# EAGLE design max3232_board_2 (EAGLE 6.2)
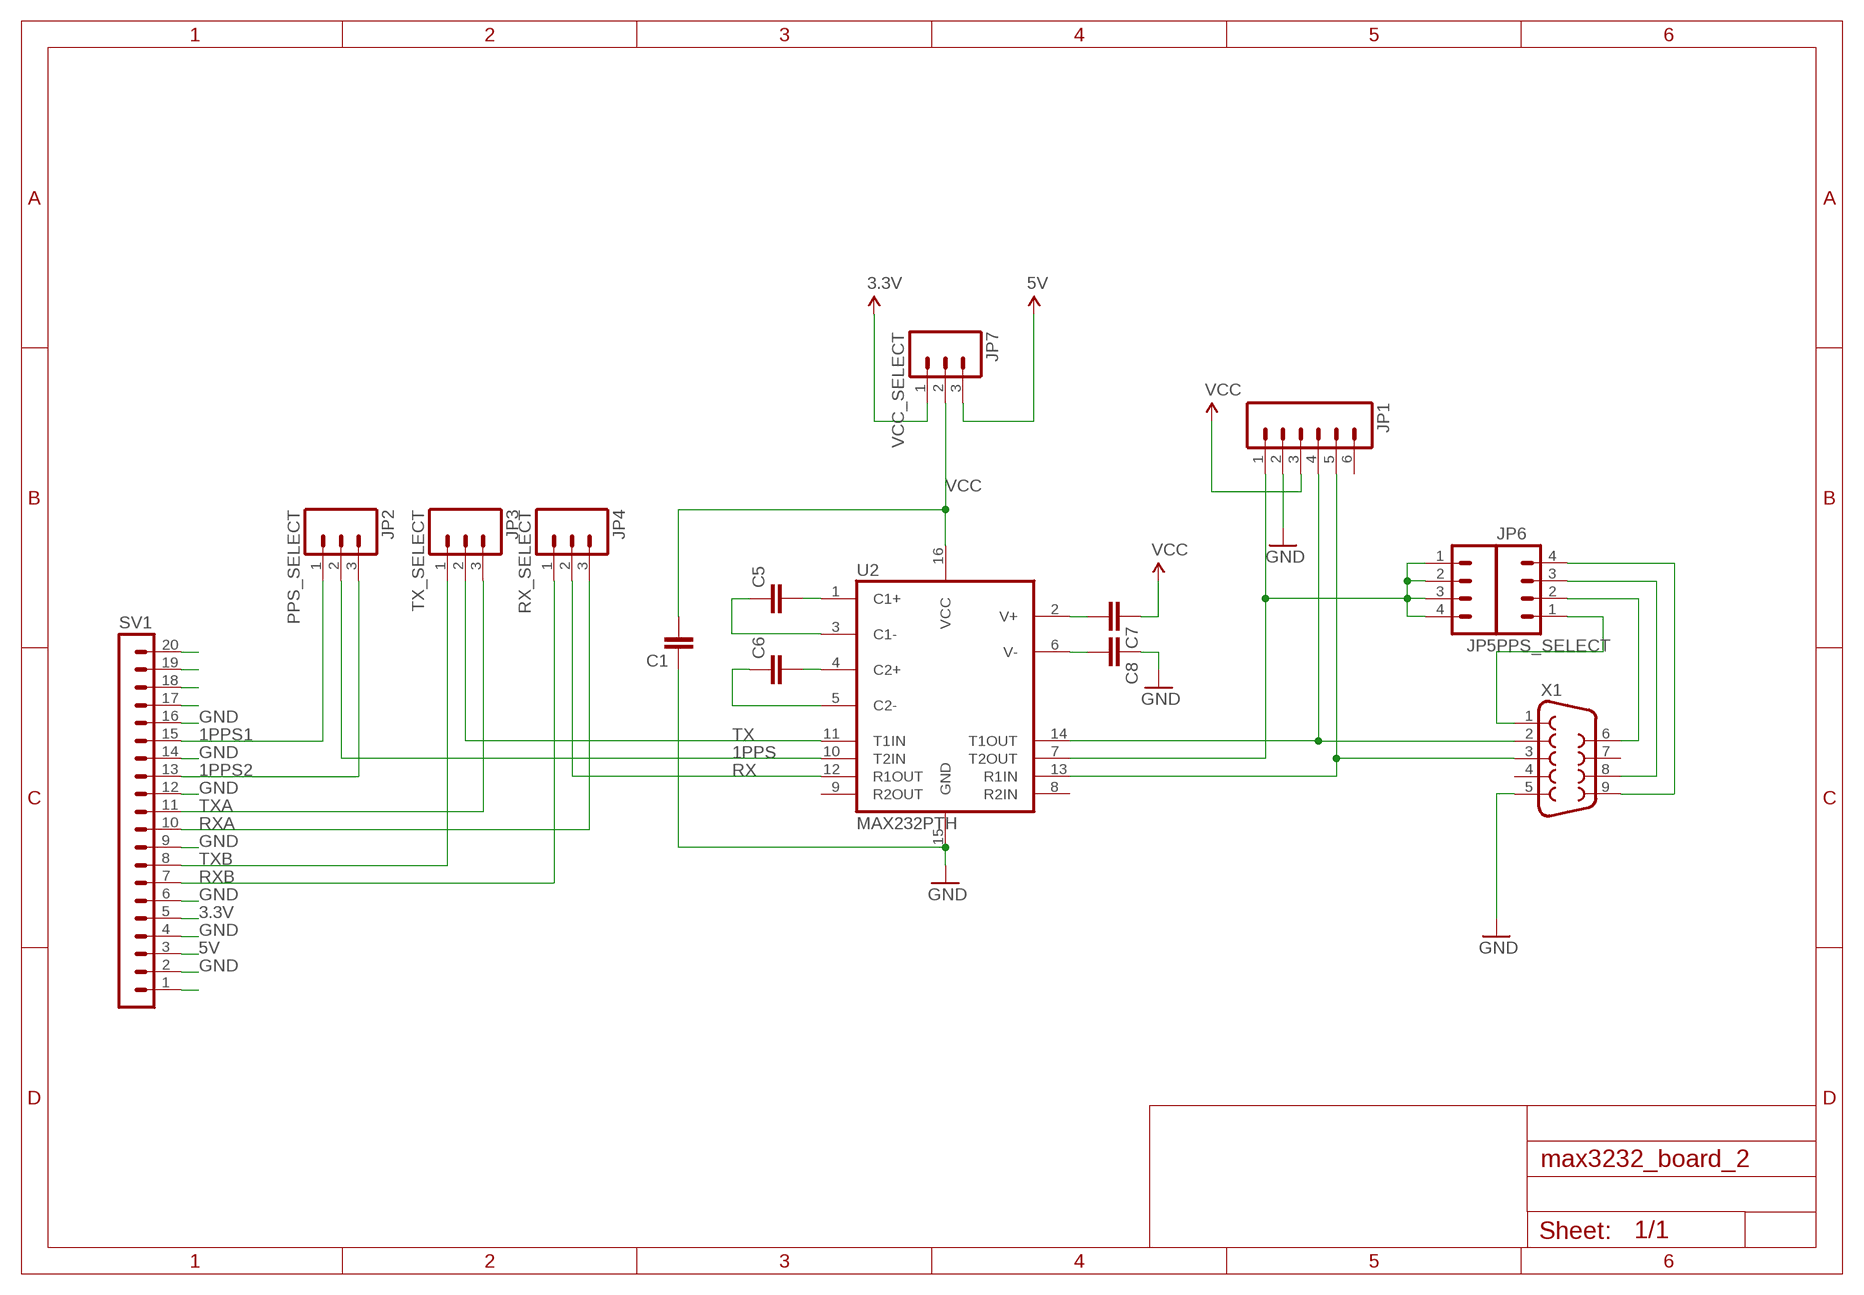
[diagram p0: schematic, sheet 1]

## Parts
C1  CAPPTH1  [CAP-PTH-5MM]
C5  CAPPTH1  [CAP-PTH-5MM]
C6  CAPPTH1  [CAP-PTH-5MM]
C7  CAPPTH1  [CAP-PTH-5MM]
C8  CAPPTH1  [CAP-PTH-5MM]
JP1  M06LONGPADS  [1X06_LONGPADS]
JP2  PPS_SELECT  M03LONGPADS  [1X03_LONGPADS]
JP3  TX_SELECT  M03LONGPADS  [1X03_LONGPADS]
JP4  RX_SELECT  M03LONGPADS  [1X03_LONGPADS]
JP5  M04PTH  [1X04]
JP6  PPS_SELECT  M04PTH  [1X04]
JP7  VСС_SELECT  M03LONGPADS  [1X03_LONGPADS]
SV1  MA20-1W  [MA20-1W]
U2  MAX232PTH  [DIL16]
X1  DB9FEMALE  [DB9]

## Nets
1PPS: JP2.2 U2.10(T2IN)
1PPS1: JP2.1 SV1.15
1PPS2: JP2.3 SV1.13
3.3V: JP7.1 SV1.5
5V: JP7.3 SV1.3
GND: C1.1 C8.1 JP1.2 SV1.2 SV1.4 SV1.6 SV1.9 SV1.12 SV1.14 SV1.16 U2.15(GND) X1.5
N$1: SV1.1
N$6: JP6.1 X1.1
N$7: JP1.4 U2.14(T1OUT) X1.2
N$8: JP1.5 U2.13(R1IN) X1.3
N$10: C6.2 U2.4(C2+)
N$11: C5.2 U2.1(C1+)
N$12: C5.1 U2.3(C1-)
N$13: C6.1 U2.5(C2-)
N$14: C8.2 U2.6(V-)
N$15: C7.2 U2.2(V+)
N$17: SV1.17
N$18: SV1.18
N$19: SV1.19
N$20: SV1.20
N$22: JP1.1 JP5.1 JP5.2 JP5.3 JP5.4 U2.7(T2OUT)
N$23: JP6.2 X1.6
N$24: JP6.3 X1.8
N$25: JP6.4 X1.9
RX: JP4.2 U2.12(R1OUT)
RXA: JP4.3 SV1.10
RXB: JP4.1 SV1.7
TX: JP3.2 U2.11(T1IN)
TXA: JP3.3 SV1.11
TXB: JP3.1 SV1.8
VCC: C1.2 C7.1 JP1.3 JP7.2 U2.16(VCC)
Unconnected: JP1.6 U2.8(R2IN) U2.9(R2OUT) X1.4 X1.7

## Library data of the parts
C1 C5-C8 = SparkFun:CAP: Capacitor
JP1 = SparkFun:M06: Header 6 Standard 6-pin 0.1" header. Use with straight break away headers (SKU : PRT-00116), right angle break away headers (PRT-00553), swiss pins (PRT-00743), machine pins (PRT-00117), and female headers (PRT-00115). Molex polarized connector foot print use with SKU : PRT-08094 with associated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
JP2-JP4 JP7 = SparkFun:M03: Header 3 Standard 3-pin 0.1" header. Use with straight break away headers (SKU : PRT-00116), right angle break away headers (PRT-00553), swiss pins (PRT-00743), machine pins (PRT-00117), and female headers (PRT-00115). Molex polarized connector foot print use with SKU : PRT-08232 with associated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
JP5 JP6 = SparkFun:M04: Header 4 Standard 4-pin 0.1" header. Use with straight break away headers (SKU : PRT-00116), right angle break away headers (PRT-00553), swiss pins (PRT-00743), machine pins (PRT-00117), and female headers (PRT-00115). Molex polarized connector foot print use with SKU : PRT-08231 with associated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
SV1 = con-lstb:MA20-1W: PIN HEADER; OC_FARNELL: unknown; OC_NEWARK: unknown
U2 = SparkFun:MAX232: RS232 Transceiver Very common IC. This is generically called 'MAX232', but works with the 3V equivalent MAX3232 generic ICs. Field tested and mother approved. Spark Fun Electronics SKU : COM-00316 (DIP) and COM-00589 (SMD)
X1 = SparkFun:DB9: DB9 Connector Standard DB9 (D-Sub 9) serial connector. Can be used for CAN bus as well as RS485 and RS232. Footprint production proven. Spark Fun Electronics SKU : PRT-00429

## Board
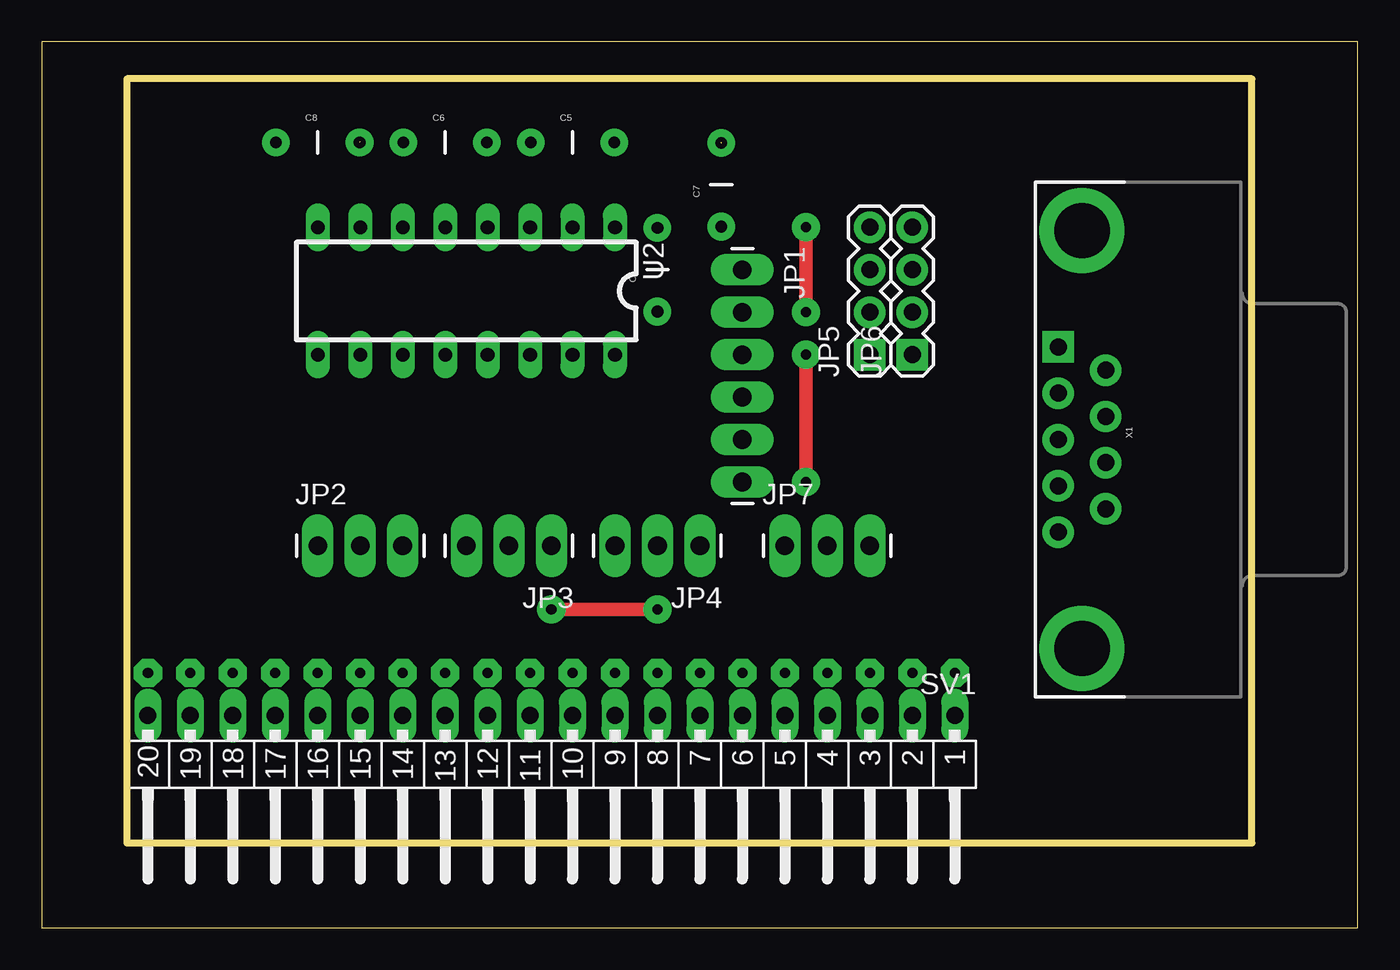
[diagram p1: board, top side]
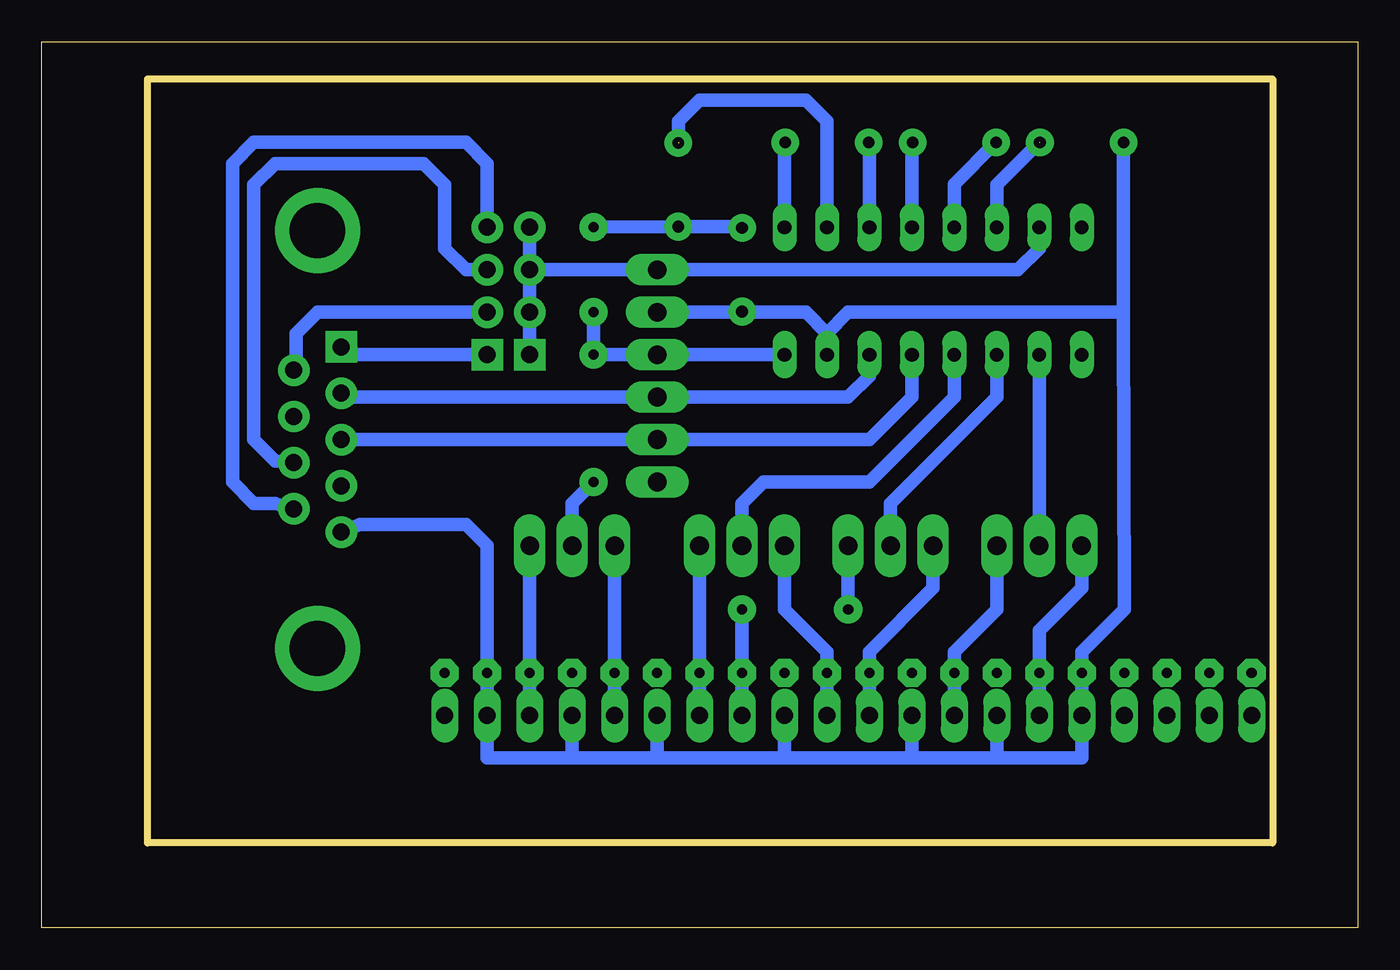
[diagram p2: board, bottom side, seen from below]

Size 78.72 x 53.01 mm. Coordinates in mm from the lower left corner, seen from the top.
Outline: 0,0 78.72,0 78.72,53.01 0,53.01 0,0
Outline: 5.08,5.08 72.39,5.08 72.39,50.8 5.08,50.8 5.08,5.08
Copper layers (1*16): Top 0.035mm / dielectric 1.5mm / Bottom 0.035mm
Design rules: minimum track width 10mil, minimum drill 24mil, track to track 8mil, track to pad 8mil, pad to pad 8mil, via to via 8mil, smd to smd 8mil, copper to edge 40mil, drill to drill 8mil, minimum pad ring 12mil, minimum via ring 12mil, stop-mask expansion 4mil, vias tented up to drill 0mil, thermal gap 10mil

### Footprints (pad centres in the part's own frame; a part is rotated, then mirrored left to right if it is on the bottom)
CAP-PTH-5MM = drill 0.7 pad 1.651: 1 -2.5,0; 2 2.5,0
1X06_LONGPADS = drill 1.118 pad 1.88 long: 1 0,0; 2 2.54,0; 3 5.08,0; 4 7.62,0; 5 10.16,0; 6 12.7,0
1X03_LONGPADS = drill 1.118 pad 1.88 long: 1 0,0; 2 2.54,0; 3 5.08,0
1X04 = drill 1.016 pad 1.88 square: 1 0,0 | drill 1.016 pad 1.88: 2 2.54,0; 3 5.08,0; 4 7.62,0
MA20-1W = drill 1.016 long: 1 -24.13,0; 2 -21.59,0; 3 -19.05,0; 4 -16.51,0; 5 -13.97,0; 6 -11.43,0; 7 -8.89,0; 8 -6.35,0; 9 -3.81,0; 10 -1.27,0; 11 1.27,0; 12 3.81,0; 13 6.35,0; 14 8.89,0; 15 11.43,0; 16 13.97,0; 17 16.51,0; 18 19.05,0; 19 21.59,0; 20 24.13,0
DIL16 = drill 0.813 long: 1 -8.89,-3.81; 2 -6.35,-3.81; 3 -3.81,-3.81; 4 -1.27,-3.81; 5 1.27,-3.81; 6 3.81,-3.81; 7 6.35,-3.81; 8 8.89,-3.81; 9 8.89,3.81; 10 6.35,3.81; 11 3.81,3.81; 12 1.27,3.81; 13 -1.27,3.81; 14 -3.81,3.81; 15 -6.35,3.81; 16 -8.89,3.81
DB9 = drill 1.016 pad 1.88 square: 1 -5.54,-1.42 | drill 1.016 pad 1.88: 2 -2.77,-1.42; 3 0,-1.42; 4 2.77,-1.42; 5 5.54,-1.42; 6 -4.15,1.42; 7 -1.38,1.42; 8 1.38,1.42; 9 4.15,1.42 | drill 3.302 pad 5.08: G1 -12.5,0; G2 12.5,0

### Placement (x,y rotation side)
C1  36.83,39.37 90 top
C5  31.75,46.99 0 top
C6  24.13,46.99 0 top
C7  40.64,44.45 90 top
C8  16.51,46.99 0 top
JP1  41.91,39.37 270 top
JP2  16.51,22.86 0 top
JP3  30.48,22.86 180 top
JP4  39.37,22.86 180 top
JP5  49.53,34.29 90 top
JP6  52.07,34.29 90 top
JP7  44.45,22.86 0 top
SV1  30.48,12.7 180 top
U2  25.4,38.1 180 top
X1  62.23,29.21 270 top

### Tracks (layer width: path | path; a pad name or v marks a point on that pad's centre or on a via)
1PPS
  Bottom 0.813: JP2.2 U2.10
1PPS1  (via drill 0.6 pad 1.68)
  Bottom 0.813: SV1.15 v19.05,15.24 19.05,17.78 16.51,20.32 JP2.1
1PPS2  (via drill 0.6 pad 1.68)
  Bottom 0.813: SV1.13 v24.13,15.24 24.13,16.51 21.59,19.05 JP2.3
3.3V  (via drill 0.6 pad 1.68)
  Bottom 0.813: SV1.5 v44.45,15.24 JP7.1
5V  (via drill 0.6 pad 1.68)
  Bottom 0.813: SV1.3 v49.53,15.24 JP7.3
GND  (via drill 0.6 pad 1.68)
  Bottom 0.813: C8.1 14.01,36.83 | 31.75,35.56 33.02,36.83 36.83,36.83 | 36.83,36.83 JP1.2 | U2.15 31.75,35.56 | 31.75,35.56 30.48,36.83 14.01,36.83 | C1.1 36.87,36.87 36.83,36.83 | 60.96,24.13 X1.5 59.69,24.13 53.34,24.13 52.07,22.86 v52.07,15.24 SV1.2 52.07,10.16 46.99,10.16 | 14.01,36.83 13.97,19.05 16.51,16.51 v16.51,15.24 SV1.16 16.51,10.16 21.59,10.16 | SV1.14 21.59,10.16 | 21.59,10.16 26.67,10.16 | SV1.12 26.67,10.16 | 26.67,10.16 34.29,10.16 | 34.29,10.16 SV1.9 | SV1.4 46.99,10.16 | 46.99,10.16 41.91,10.16 | SV1.6 41.91,10.16 | 41.91,10.16 34.29,10.16
N$2  (via drill 0.6 pad 1.68)
  other vias: 6.35,15.24
N$3  (via drill 0.6 pad 1.68)
  other vias: 8.89,15.24
N$4  (via drill 0.6 pad 1.68)
  other vias: 11.43,15.24
N$5  (via drill 0.6 pad 1.68)
  other vias: 13.97,15.24
N$6
  Bottom 0.813: JP6.1 60.35,34.29 X1.1
N$7
  Bottom 0.813: U2.14 29.21,33.02 30.48,31.75 JP1.4 60.58,31.75 X1.2
N$8
  Bottom 0.813: U2.13 26.67,31.75 29.21,29.21 JP1.5 X1.3
N$9  (via drill 0.6 pad 1.68)
  other vias: 21.59,15.24
N$10
  Bottom 0.813: U2.4 26.67,46.95 C6.2
N$11
  Bottom 0.813: U2.1 34.29,46.95 C5.2
N$12
  Bottom 0.813: U2.3 29.21,46.95 C5.1
N$13
  Bottom 0.813: U2.5 24.13,44.49 C6.1
N$14  (1 unrouted)
  Bottom 0.813: U2.6 21.59,44.45 19.05,46.99
N$15  (1 unrouted)
  Bottom 0.813: U2.2 31.75,48.26 33.02,49.53 39.37,49.53 40.64,48.26 40.64,46.99
N$16  (via drill 0.6 pad 1.68)
  other vias: 26.67,15.24
N$21  (via drill 0.6 pad 1.68)
  other vias: 34.29,15.24
N$22
  Bottom 0.813: U2.7 19.05,40.64 20.32,39.37 JP1.1 JP5.3 | JP5.1 JP5.2 JP5.3 | JP5.3 JP5.4
N$23
  Bottom 0.813: JP6.2 62.23,36.83 63.5,35.56 63.5,33.51 X1.6
N$24
  Bottom 0.813: JP6.3 53.34,39.37 54.61,40.64 54.61,44.45 55.88,45.72 64.77,45.72 66.04,44.45 66.04,29.21 64.77,27.94 X1.8
N$25
  Bottom 0.813: JP6.4 52.07,45.72 53.34,46.99 66.04,46.99 67.31,45.72 67.31,26.67 66.04,25.4 64.77,25.4 X1.9
N$26  (via drill 0.6 pad 1.68)
  other vias: 41.91,15.24
N$27  (via drill 0.6 pad 1.68)
  other vias: 46.99,15.24
N$28  (via drill 0.6 pad 1.68)
  other vias: 54.61,15.24
RX
  Bottom 0.813: U2.12 24.13,31.75 29.21,26.67 35.56,26.67 36.83,25.4 JP4.2
RXA  (via drill 0.6 pad 1.68)
  Bottom 0.813: SV1.10 v31.75,15.24 31.75,16.51 34.29,19.05 JP4.3
RXB  (via drill 0.6 pad 1.68)
  Bottom 0.813: SV1.7 v39.37,15.24 JP4.1
TX
  Bottom 0.813: JP3.2 27.94,25.4 21.59,31.75 U2.11
TXA  (via drill 0.6 pad 1.68)
  Bottom 0.813: SV1.11 v29.21,15.24 29.21,16.51 25.4,20.32 JP3.3
TXB  (via drill 0.6, 0.6 pad 1.68)
  Top 0.813: v36.83,19.05 v30.48,19.05
  Bottom 0.813: SV1.8 v36.83,15.24 v36.83,19.05 | v30.48,19.05 JP3.1
VCC  (via drill 0.6, 0.6 pad 1.68)
  Top 0.813: v45.72,26.67 v45.72,34.29 | v45.72,36.83 v45.72,41.91
  Bottom 0.813: U2.16 JP1.3 v45.72,34.29 v45.72,36.83 | C1.2 36.91,41.95 C7.1 v45.72,41.91 | JP7.2 46.99,25.4 v45.72,26.67

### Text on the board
_tNames: C8 | C6 | C5 | C7 | U2 | JP1 | C1 | JP5 | JP6 | X1 | JP2 | JP7 | JP3 | JP4 | SV1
